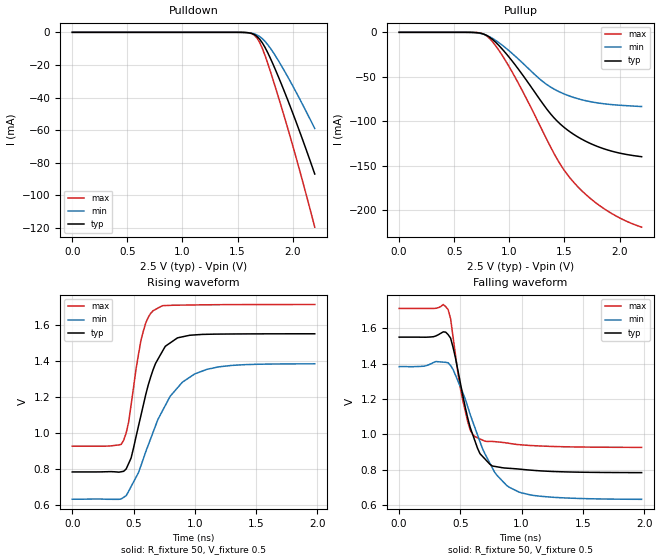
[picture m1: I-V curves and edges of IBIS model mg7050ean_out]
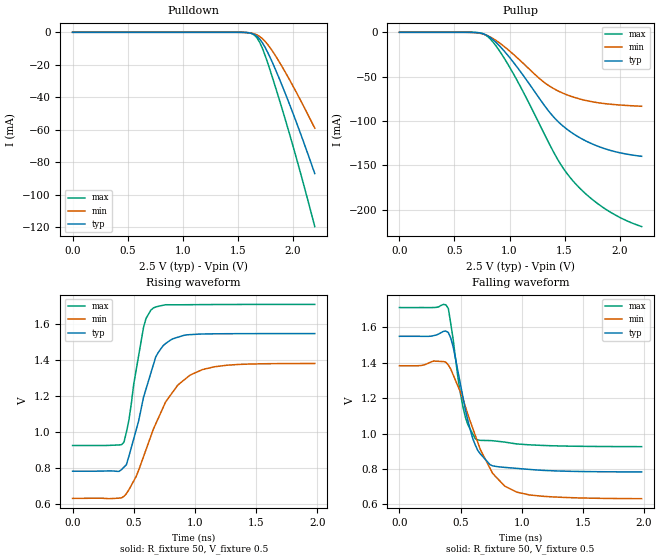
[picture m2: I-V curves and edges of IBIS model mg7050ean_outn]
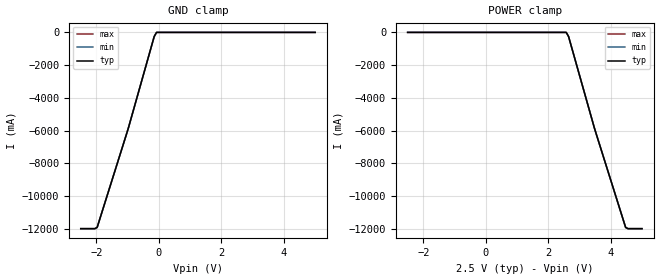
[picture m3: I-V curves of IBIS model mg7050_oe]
|   IBIS File mg7050ean_4out_25v.ibs
[IBIS Ver]   3.2
[Comment Char]   |_char
[File name]   mg7050ean_4out_25v.ibs
[File Rev]   1.0
[Date]   Aug 02, 2013
[Source]
|   Component MG7050EAN LV-PECL 4-OUTPUT 2.5V
[Component]   mg7050ean-pecl-4out
[Manufacturer]   Seiko Epson Corporation
[Package]
| variable   typ   min   max
R_pkg   0.27   NA   NA
L_pkg   1.66n   NA   NA
C_pkg   0.53p   NA   NA
[Pin]   signal_name   model_name   R_pin   L_pin   C_pin
1   vcc1   POWER   NA   NA   NA
2   out1p   mg7050ean_out   0.34   2.1nH   0.58pF
3   out1n   mg7050ean_outn  0.25   1.5nH   0.50pF
4   out2p   mg7050ean_out   0.22   1.3nH   0.44pF
5   out2n   mg7050ean_outn  0.25   1.7nH   0.59pF
6   fsel   mg7050_fsel   NA   NA   NA
7   oe   mg7050_oe   NA   NA   NA
8   out3n   mg7050ean_outn  0.25   1.7nH   0.62pF
9   out3p   mg7050ean_out   0.22   1.3nH   0.49pF
10   out4n   mg7050ean_outn  0.25   1.5nH   0.46pF
11   out4p   mg7050ean_out   0.34   2.1nH   0.57pF
12   vcc2   POWER   NA   NA   NA
13   vcc   POWER   NA   NA   NA
14   gnd   GND   NA   NA   NA
[Diff Pin] inv_pin vdiff   tdelay_typ
2   3   0   0
4   5   0   0
9   8   0   0
11   10   0   0
| Models and submodels in the file (4): mg7050ean_out (Output_ECL), mg7050ean_outn (Output_ECL), mg7050_oe (Input), mg7050_fsel (Input)
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[Model]   mg7050ean_out
Model_type Output_ECL
Enable Active-High
Polarity Non-Inverting
Vref=0.5
Vmeas=1.17
Rref=50
Cref=0
C_comp   0.121p   0.121p   0.121p
[Temperature Range] 25   90   -40
[Voltage Range]   2.5   2.375   2.625
[Pullup Reference]  2.5   2.375   2.625
[Pulldown Reference]2.5   2.375   2.625
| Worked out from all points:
|   falling waveform, R_fixture 50, V_fixture 0.5: 20-80 % time 162ps typ, 262ps min, 117ps max; typ from 1.55 V to 0.784 V
|   rising waveform, R_fixture 50, V_fixture 0.5: 20-80 % time 182ps typ, 296ps min, 111ps max; typ from 0.783 V to 1.55 V
[Pullup]
0V        299.6pA    407.8pA    314.4pA
700mV     -323.5uA   -552.1uA   -202.9uA
800mV     -3.877mA   -3.779mA   -4.606mA
875mV     -11.1mA    -9.029mA   -14.96mA
1V        -28.31mA   -21.02mA   -39.12mA
1.375V    -91.8mA    -61.58mA   -129.1mA
1.475V    -104.6mA   -68.07mA   -150.9mA
1.55V     -111.9mA   -71.76mA   -163.6mA
1.7V      -122.9mA   -77.03mA   -183mA
1.85V     -130.6mA   -80.18mA   -197.5mA
2.025V    -136.4mA   -82.15mA   -210.1mA
2.2V      -139.8mA   -83.4mA    -219mA
[Pulldown]
0V        299.7pA    407.7pA    314.4pA
1.55V     -60.83uA   -73.05uA   -33.15uA
1.6V      -310uA     -275.3uA   -272.2uA
1.65V     -1.317mA   -925.3uA   -1.635mA
1.675V    -2.45mA    -1.59mA    -3.401mA
1.7V      -4.18mA    -2.583mA   -6.195mA
1.725V    -6.526mA   -3.943mA   -9.951mA
1.775V    -12.7mA    -7.704mA   -19.34mA
1.825V    -20.08mA   -12.5mA    -29.84mA
2V        -49.43mA   -32.8mA    -69.43mA
2.1V      -67.73mA   -45.63mA   -93.86mA
2.2V      -86.89mA   -58.96mA   -119.5mA
[Falling Waveform]
R_fixture=50
V_fixture=0.5
V_fixture_min=0.375
V_fixture_max=0.625
0s        1.55V      1.383V     1.712V
400ps     1.564V     1.405V     1.705V
440ps     1.492V     1.368V     1.552V
520ps     1.219V     1.235V     1.191V
580ps     1.04V      1.113V     1.024V
620ps     960.9mV    1.035V     986.9mV
660ps     891mV      958.6mV    974.3mV
780ps     819.1mV    785.5mV    958.9mV
980ps     803.8mV    673.5mV    942mV
1.98ns    783.8mV    632.9mV    926.5mV
[Rising Waveform]
R_fixture=50
V_fixture=0.5
V_fixture_min=0.375
V_fixture_max=0.625
0s        783.4mV    632.1mV    926.3mV
400ps     784.6mV    633.8mV    936.7mV
460ps     829.8mV    676.1mV    1.059V
560ps     1.095V     816.5mV    1.511V
600ps     1.212V     895.7mV    1.61V
660ps     1.35V      1.004V     1.677V
760ps     1.48V      1.153V     1.706V
1ns       1.543V     1.327V     1.709V
1.3ns     1.548V     1.374V     1.711V
1.98ns    1.549V     1.383V     1.712V
[Ramp]
R_load=50
dV/dt_r   4.596E-1/1.825E-10   4.506E-1/2.953E-10   4.713E-1/1.122E-10
dV/dt_f   4.597E-1/1.625E-10   4.506E-1/2.626E-10   4.713E-1/1.166E-10
|[End   mg7050ean_out
[Model]   mg7050ean_outn
Model_type Output_ECL
Enable Active-High
Polarity Inverting
Vref=0.5
Vmeas=1.17
Rref=50
Cref=0
C_comp   0.121p   0.121p   0.121p
[Temperature Range] 25   90   -40
[Voltage Range]   2.5   2.375   2.625
[Pullup Reference]  2.5   2.375   2.625
[Pulldown Reference]2.5   2.375   2.625
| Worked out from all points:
|   falling waveform, R_fixture 50, V_fixture 0.5: 20-80 % time 153ps typ, 257ps min, 109ps max; typ from 1.55 V to 0.784 V
|   rising waveform, R_fixture 50, V_fixture 0.5: 20-80 % time 181ps typ, 292ps min, 109ps max; typ from 0.783 V to 1.55 V
[Pullup]
0V        299.6pA    407.8pA    314.4pA
700mV     -323.5uA   -552.1uA   -202.9uA
800mV     -3.877mA   -3.779mA   -4.606mA
875mV     -11.1mA    -9.029mA   -14.96mA
1V        -28.31mA   -21.02mA   -39.12mA
1.375V    -91.8mA    -61.58mA   -129.1mA
1.475V    -104.5mA   -68.07mA   -150.9mA
1.55V     -111.9mA   -71.76mA   -163.6mA
1.7V      -122.9mA   -77.03mA   -183mA
1.85V     -130.6mA   -80.17mA   -197.5mA
2.025V    -136.4mA   -82.15mA   -210.1mA
2.2V      -139.8mA   -83.4mA    -219mA
[Pulldown]
0V        299.7pA    407.8pA    314.4pA
1.55V     -60.83uA   -73.05uA   -33.15uA
1.6V      -310uA     -275.3uA   -272.2uA
1.65V     -1.317mA   -925.3uA   -1.635mA
1.675V    -2.45mA    -1.59mA    -3.401mA
1.7V      -4.18mA    -2.583mA   -6.195mA
1.725V    -6.526mA   -3.943mA   -9.951mA
1.775V    -12.7mA    -7.704mA   -19.34mA
1.825V    -20.08mA   -12.5mA    -29.84mA
2V        -49.43mA   -32.8mA    -69.43mA
2.1V      -67.73mA   -45.62mA   -93.86mA
2.2V      -86.89mA   -58.96mA   -119.5mA
[Falling Waveform]
R_fixture=50
V_fixture=0.5
V_fixture_min=0.375
V_fixture_max=0.625
0s        1.55V      1.383V     1.712V
400ps     1.57V      1.387V     1.706V
440ps     1.487V     1.331V     1.529V
480ps     1.345V     1.265V     1.308V
520ps     1.203V     1.195V     1.148V
560ps     1.072V     1.107V     1.049V
620ps     936.2mV    990mV      971.2mV
760ps     818.5mV    778.2mV    960.2mV
960ps     803.7mV    669.7mV    941.8mV
1.98ns    783.8mV    632.8mV    926.6mV
[Rising Waveform]
R_fixture=50
V_fixture=0.5
V_fixture_min=0.375
V_fixture_max=0.625
0s        783.4mV    632.1mV    926.3mV
420ps     805.9mV    643.7mV    944.6mV
460ps     864.7mV    679.3mV    1.065V
500ps     963.6mV    729.1mV    1.268V
580ps     1.195V     864.2mV    1.583V
660ps     1.374V     1.016V     1.691V
740ps     1.482V     1.138V     1.707V
860ps     1.529V     1.262V     1.71V
1.06ns    1.547V     1.349V     1.711V
1.98ns    1.549V     1.383V     1.712V
[Ramp]
R_load=50
dV/dt_r   4.596E-1/1.728E-10   4.506E-1/2.903E-10   4.713E-1/1.082E-10
dV/dt_f   4.596E-1/1.536E-10   4.506E-1/2.575E-10   4.713E-1/1.092E-10
|[End   mg7050ean_outn
[Model]   mg7050_oe
Model_type Input
Vinh=1.75
Vinl=0.75
C_comp   3p   3p   3p
[Temperature Range] 25   90   -40
[Voltage Range]   2.5   2.375   2.625
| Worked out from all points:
|   GND clamp passes 1 mA (typ) near -0.08 V on its own axis
[GND Clamp]
-2.5V     -12A       -12A       -12A
-2.05V    -12A       -12A       -12A
-1.975V   -11.92A    -11.92A    -11.92A
-975mV    -5.84A     -5.84A     -5.84A
-150mV    -254mA     -254mA     -254mA
-75mV     -24.98uA   -21.67uA   -29.1uA
5V        24.28uA    23.28uA    25.61uA
[POWER Clamp]
-2.5V     24.28uA    23.28uA    25.61uA
2.575V    -24.98uA   -21.67uA   -29.1uA
2.65V     -254mA     -254mA     -254mA
3.475V    -5.84A     -5.84A     -5.84A
4.475V    -11.92A    -11.92A    -11.92A
4.55V     -12A       -12A       -12A
5V        -12A       -12A       -12A
